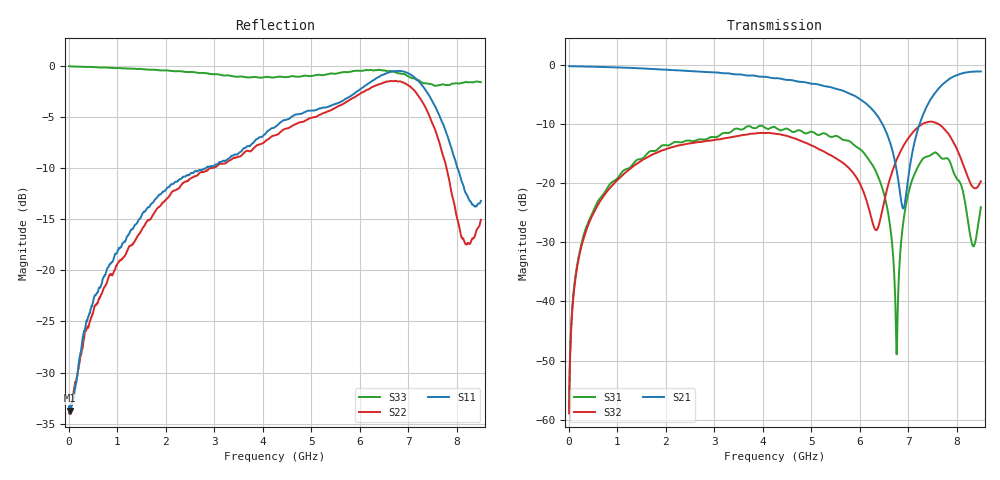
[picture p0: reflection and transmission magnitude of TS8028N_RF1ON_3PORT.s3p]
!Created with skrf (http://scikit-rf.org).
# GHz S RI R 50.0
!freq ReS11 ImS11 ReS12 ImS12 ReS13 ImS13
! ReS21 ImS21 ReS22 ImS22 ReS23 ImS23
! ReS31 ImS31 ReS32 ImS32 ReS33 ImS33
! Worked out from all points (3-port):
!   1601 points, 10 MHz to 8.5 GHz, reference 50 ohm
!   strongest paths, dB at 10 MHz, 2.132 GHz, 4.255 GHz, 6.378 GHz, 8.5 GHz:
!     S21: -0.2, -0.9, -2.3, -8.7, -1.1
!     S32: -58.9, -13.9, -11.6, -27.6, -19.7
!     S31: -58.2, -13.3, -10.5, -18.8, -24.1
!   lowest |S11| = -33.7 dB at 31.23 MHz (marker M1), VSWR 1.04, Z = 52 - j0.471 ohm
!   |S11| at or under -10 dB: start of sweep to 2.827 GHz; 8.019 GHz to end of sweep
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0.01  0.0214 -0.00103  0.9741 -0.00569  0.000198 0.0012
      0.9742 -0.00575  0.02 -0.00044  0.000188 0.00114
      0.000182 0.00121  0.000178 0.00112  0.998 -0.00942
0.031225  0.0201 -0.00452  0.9733 -0.0131  0.000263 0.0037
          0.9733 -0.013  0.0211 -0.00389  0.000303 0.0035
          0.000266 0.00372  0.000306 0.00352  0.9957 -0.0243
0.243475  0.0131 -0.0372  0.9641 -0.0956  0.0043 0.028
          0.9645 -0.0955  0.0174 -0.0337  0.00477 0.0265
          0.00431 0.028  0.00477 0.0266  0.9753 -0.1802
0.8643063  -0.0144 -0.1072  0.9004 -0.3175  0.0487 0.0869
           0.9005 -0.3175  -0.03 -0.0911  0.0502 0.0777
           0.0488 0.0868  0.0503 0.0776  0.7936 -0.5739
2.546387  -0.1975 -0.226  0.4986 -0.7304  0.2246 0.0257
          0.4989 -0.7311  -0.2716 -0.0847  0.2172 -0.0225
          0.2244 0.0255  0.2169 -0.0226  -0.1434 -0.9239
4.255  -0.4697 -0.1797  -0.0362 -0.7702  0.2014 -0.2184
       -0.0378 -0.7704  -0.357 0.2871  0.1132 -0.2369
       0.2011 -0.2194  0.1139 -0.2365  -0.8406 -0.2636
6.637506  -0.7172 0.5998  -0.2066 -0.0561  -0.037 -0.0165
          -0.2067 -0.0563  0.5578 0.6345  0.0936 -0.0641
          -0.037 -0.0166  0.0934 -0.064  0.0913 0.9401
6.764856  -0.6484 0.6881  -0.1201 -0.0428  0.00118 -0.00335
          -0.1198 -0.0424  0.6386 0.5505  0.123 -0.0995
          0.00117 -0.00338  0.1235 -0.0998  0.2088 0.9022
7.290175  -0.1869 0.7802  0.197 -0.3054  0.1004 -0.1222
          0.1966 -0.3067  0.6689 -0.0141  0.0567 -0.3103
          0.1003 -0.1223  0.0574 -0.3102  0.6419 0.5226
8.5  -0.1018 0.1936  -0.5907 -0.6508  0.0407 0.0477
     -0.5918 -0.6503  -0.1189 0.1307  -0.00904 -0.1032
     0.0406 0.0476  -0.00849 -0.1033  0.2831 -0.7841
